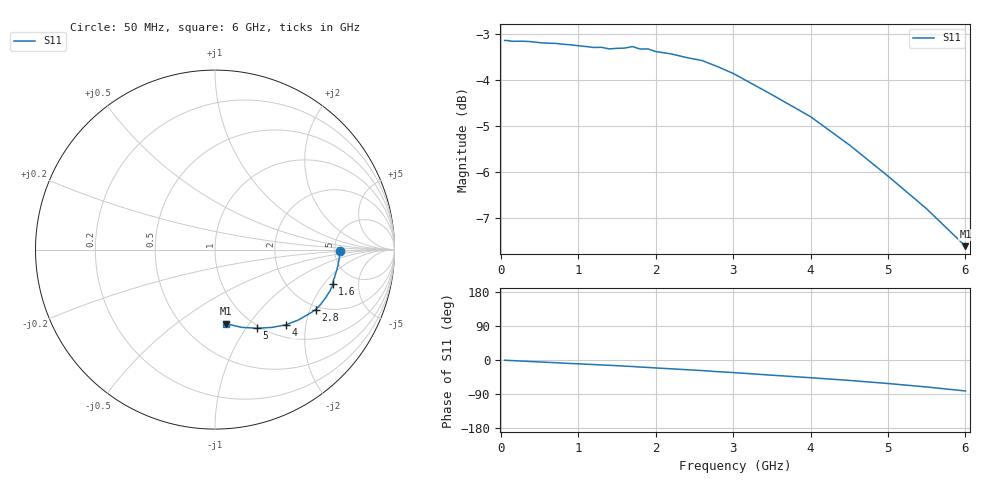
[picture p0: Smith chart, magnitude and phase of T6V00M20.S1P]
! SIEMENS Discrete & RF Semiconductors
! BAT62
! Si Schottky Diode in SOT143
! IF = 0.2 mA
! S-Parameters:  February  1997
# GHz  S  MA  R  50
!  f  S11
! GHz  MAG  ANG
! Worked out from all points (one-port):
!   34 points, 50 MHz to 6 GHz, reference 50 ohm
!   lowest |S11| = -7.6 dB at 6 GHz (marker M1), VSWR 2.43, Z = 39.2 - j39.2 ohm
!   |S11| at or under -10 dB: nowhere
!   S11 on the Smith chart (normalised r, x): 50 MHz: 5.58, -0.16; 1.6 GHz: 3.45, -2.46; 2.8 GHz: 1.88, -2.19; 4 GHz: 1.23, -1.55; 5 GHz: 0.97, -1.12; 6 GHz: 0.78, -0.78
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0.05  0.6961 -0.6
0.3  0.6947 -3.1
0.4  0.6939 -4.2
0.5  0.6923 -5.1
0.7  0.6911 -7.1
0.8  0.6896 -8.1
0.9  0.6885 -9.2
1  0.687 -10.0
1.1  0.6856 -11.1
1.2  0.684 -12.0
1.3  0.6843 -13.1
1.4  0.6816 -13.9
1.6  0.6829 -16.2
1.7  0.6855 -17.2
1.8  0.6813 -18.6
1.9  0.6815 -19.6
2  0.6771 -21.0
2.2  0.6731 -23.2
2.4  0.667 -25.6
2.6  0.6621 -27.9
2.8  0.6521 -30.8
3  0.6412 -33.1
3.5  0.6082 -40.1
4  0.5757 -46.7
4.5  0.5366 -53.9
5  0.4964 -62.0
5.5  0.4575 -71.2
6  0.4169 -81.7
